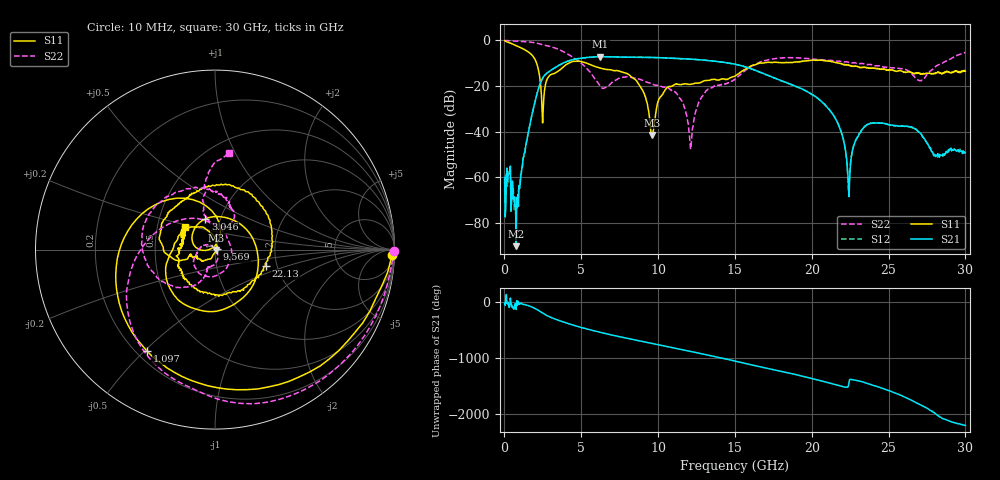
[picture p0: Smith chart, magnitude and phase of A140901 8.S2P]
!  2-Port S-parameters saved by WinCal
! VAR MeasName=S-Parameters (CALIBRATED_DATA) read from VNA (N5244A)
! VAR MeasDate=11/3/2014 9:27:12 AM
! VAR NAME=A140901 8
! VAR FILENAME=A140901 8.S2P
! VAR DATE=11/3/2014 9:27:12 AM
! VAR PHYS_PORTS=1,2
# Hz S RI R 50
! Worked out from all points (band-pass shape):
!   801 points, 10 MHz to 30 GHz, reference 50 ohm
!   highest |S21| = -7.13 dB at 6.233 GHz (marker M1); lowest = -90.2 dB at 759.8 MHz (marker M2)
!   |S21| within 3 dB of the highest: 3.765 GHz to 14.76 GHz (11 GHz wide, 119 % of centre)
!   lowest |S11| = -41.5 dB at 9.607 GHz (marker M3), VSWR 1.02, Z = 50.8 - j0.134 ohm
!   |S11| at or under -10 dB: 2.093 GHz to 4.192 GHz (2.099 GHz wide, 66.8 % of centre); 5.351 GHz to 16.61 GHz (11.26 GHz wide, 103 % of centre); 21.76 GHz to end of sweep
!   |S22| runs from -47.7 to 0.0 dB; largest |S21 - S12| = 0.0033
!   S11 on the Smith chart (normalised r, x): 10 MHz: 23, -55; 1.097 GHz: 0.24, -0.51; 3.046 GHz: 0.85, +0.30; 9.569 GHz: 1.02, +0.00; 22.13 GHz: 1.75, -0.35; 30 GHz: 0.69, +0.18
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1e7  0.9866 -0.0304  0.000978 -0.000203  -1.61e-05 -0.000549  0.9958 -0.00863
7.5975e8  0.0126 -0.7695  -1.77e-05 -2.52e-05  2.88e-06 0.000129  0.8495 -0.4531
1.097138e9  -0.3775 -0.5669  0.00118 -0.000422  0.00115 -0.000384  0.7231 -0.6149
2.034325e9  -0.2106 0.2866  -0.0212 -0.048  -0.0212 -0.0478  0.1986 -0.8586
2.484175e9  -0.00958 0.0122  -0.1457 0.0286  -0.1454 0.0283  -0.0666 -0.801
3.046488e9  -0.0546 0.1706  0.00254 0.2244  0.00221 0.2238  -0.3254 -0.647
5.033325e9  -0.229 -0.2524  -0.00895 -0.4092  -0.00943 -0.4096  -0.2801 0.1304
6.232925e9  -0.2456 -0.0171  -0.4388 -0.0294  -0.4386 -0.0293  0.0617 0.0773
8.55715e9  -0.0584 0.1212  0.3094 0.295  0.3091 0.2952  -0.1134 -0.0921
9.569312e9  0.00933 0.00136  0.4097 -0.1049  0.409 -0.104  -0.1076 -0.0322
9.6068e9  0.00834 -0.00132  0.4052 -0.1197  0.4046 -0.1186  -0.1078 -0.0309
1.001916e10  -0.0186 -0.0439  0.3216 -0.269  0.3215 -0.2683  -0.1026 -0.0189
1.148118e10  -0.1002 -0.0397  -0.215 -0.3341  -0.2149 -0.3342  -0.0423 0.0273
1.211846e10  -0.1025 -0.0355  -0.3627 -0.1373  -0.3628 -0.1371  0.00354 0.00213
1.305565e10  -0.1236 -0.0442  -0.3052 0.205  -0.3037 0.2061  0.00456 -0.0724
1.5005e10  -0.157 -0.0526  0.2659 0.1392  0.2663 0.1366  -0.0488 -0.1334
2.002832e10  0.0584 0.365  0.0184 0.0623  0.0181 0.0627  -0.2345 0.3079
2.212762e10  0.2833 -0.0912  0.00124 -0.00514  0.00118 -0.00497  -0.0308 0.3374
2.242752e10  0.2423 -0.1566  0.000365 8.48e-05  0.000523 0.00029  -0.0173 0.3288
2.336471e10  0.04 -0.2555  0.0118 0.00186  0.0122 0.0018  0.0413 0.3069
2.501416e10  -0.1904 -0.1089  -0.011 -0.00867  -0.0112 -0.00869  0.0838 0.2438
3e10  -0.1686 0.1265  0.00243 -0.00249  0.00231 -0.0025  0.0776 0.5389
